FUNCTION_BLOCK FB17
TITLE =Set Encoder Parameter
//*****************************************************************************
//* maxon motor ag
//* R&D
//* all rights reserved
//*****************************************************************************
//* Summary:  Set encoder parameter
//*
//* Remarks:
//*
//* Created under: STEP7 REV5.2+SP1
//*****************************************************************************
//* History:
//* 18.05.2004 | INA   first release
//*
//*
//*****************************************************************************
//

AUTHOR:INA
FAMILY:Configur
NAME:SEncPara
VERSION:00.01


VAR_INPUT

Write : BOOL //A rising edge start the command

  NodeID : BYTE //Adress of the maxon device

  Counts : WORD //Incremental Encoder Counts

  PositionSensorType : WORD //Position Sensor Type

END_VAR
VAR_OUTPUT
  Done : BOOL //Data valid flag is TRUE if data were available

  Err : BOOL //Error flag is TRUE if an Error has occured, see ErrNo for more details

  ErrNo : DINT //Contains detailed error information

END_VAR
VAR
  xEdgeMerker : BOOL //Edge Merker

  xEdgeFlag : BOOL //Edge Flag

  xStep : INT
END_VAR

BEGIN

NETWORK
TITLE = Activate the service function
//

// SDO Write "Set Encoder Parameter"

       U    #Write
       FP   #xEdgeFlag                   // recognize a positiv edge of the Read signal
       =    #xEdgeMerker                 // and set the xEdgeMerker for one cycle to true

       L    #xStep
       L    0
       ==I
       U    #xEdgeMerker
       SPB  nstp                         // iStep = 1 -> fnc1

       L    #xStep                       // jump list
       SPL  List
       SPA  rdef
       SPA  fnc1
       SPA  fncE
List  :SPA  rdef

rdef  :NOP  0
       R    #Done                        // reset Done
       R    #Err
       L    0
       T    #xStep                       // iStep = 0
       SPA  end

fnc1  :NOP  0
       CALL FC15
         NodeID:=#NodeID
         Index:=DW#16#00002210
         SubIndex:=DW#16#00000001
         ValueIn:=#Counts
         RET_VAL:=#Done
         Err:=#Err
         ErrNo:=#ErrNo

       L    1
       U    #Err
       SPB  fncE

       NOP  0
       CALL FC15
         NodeID:=#NodeID
         Index:=DW#16#00002210
         SubIndex:=DW#16#00000002
         ValueIn:=#PositionSensorType
         RET_VAL:=#Done
         Err:=#Err
         ErrNo:=#ErrNo

fncE  :NOP  0
       L    0
       T    #xStep
       SPA  end

nstp  :NOP  0
       L    #xStep
       INC            1
       T    #xStep

end   :NOP  0
END_FUNCTION_BLOCK
